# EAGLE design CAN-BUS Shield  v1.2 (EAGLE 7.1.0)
DESCRIPTION: microOBD 200 OBD-II Module; HW_REV: 1.4; PCB_REV: C; PCB_SPEC1: Layer Count: 4; PCB_SPEC2: Size: 1.3" x 0.59"; PCB_SPEC3: Finish Thickness: 0.049" - 0.052"; PCB_SPEC4: Copper Weight: 1oz; TITLE: STM1120

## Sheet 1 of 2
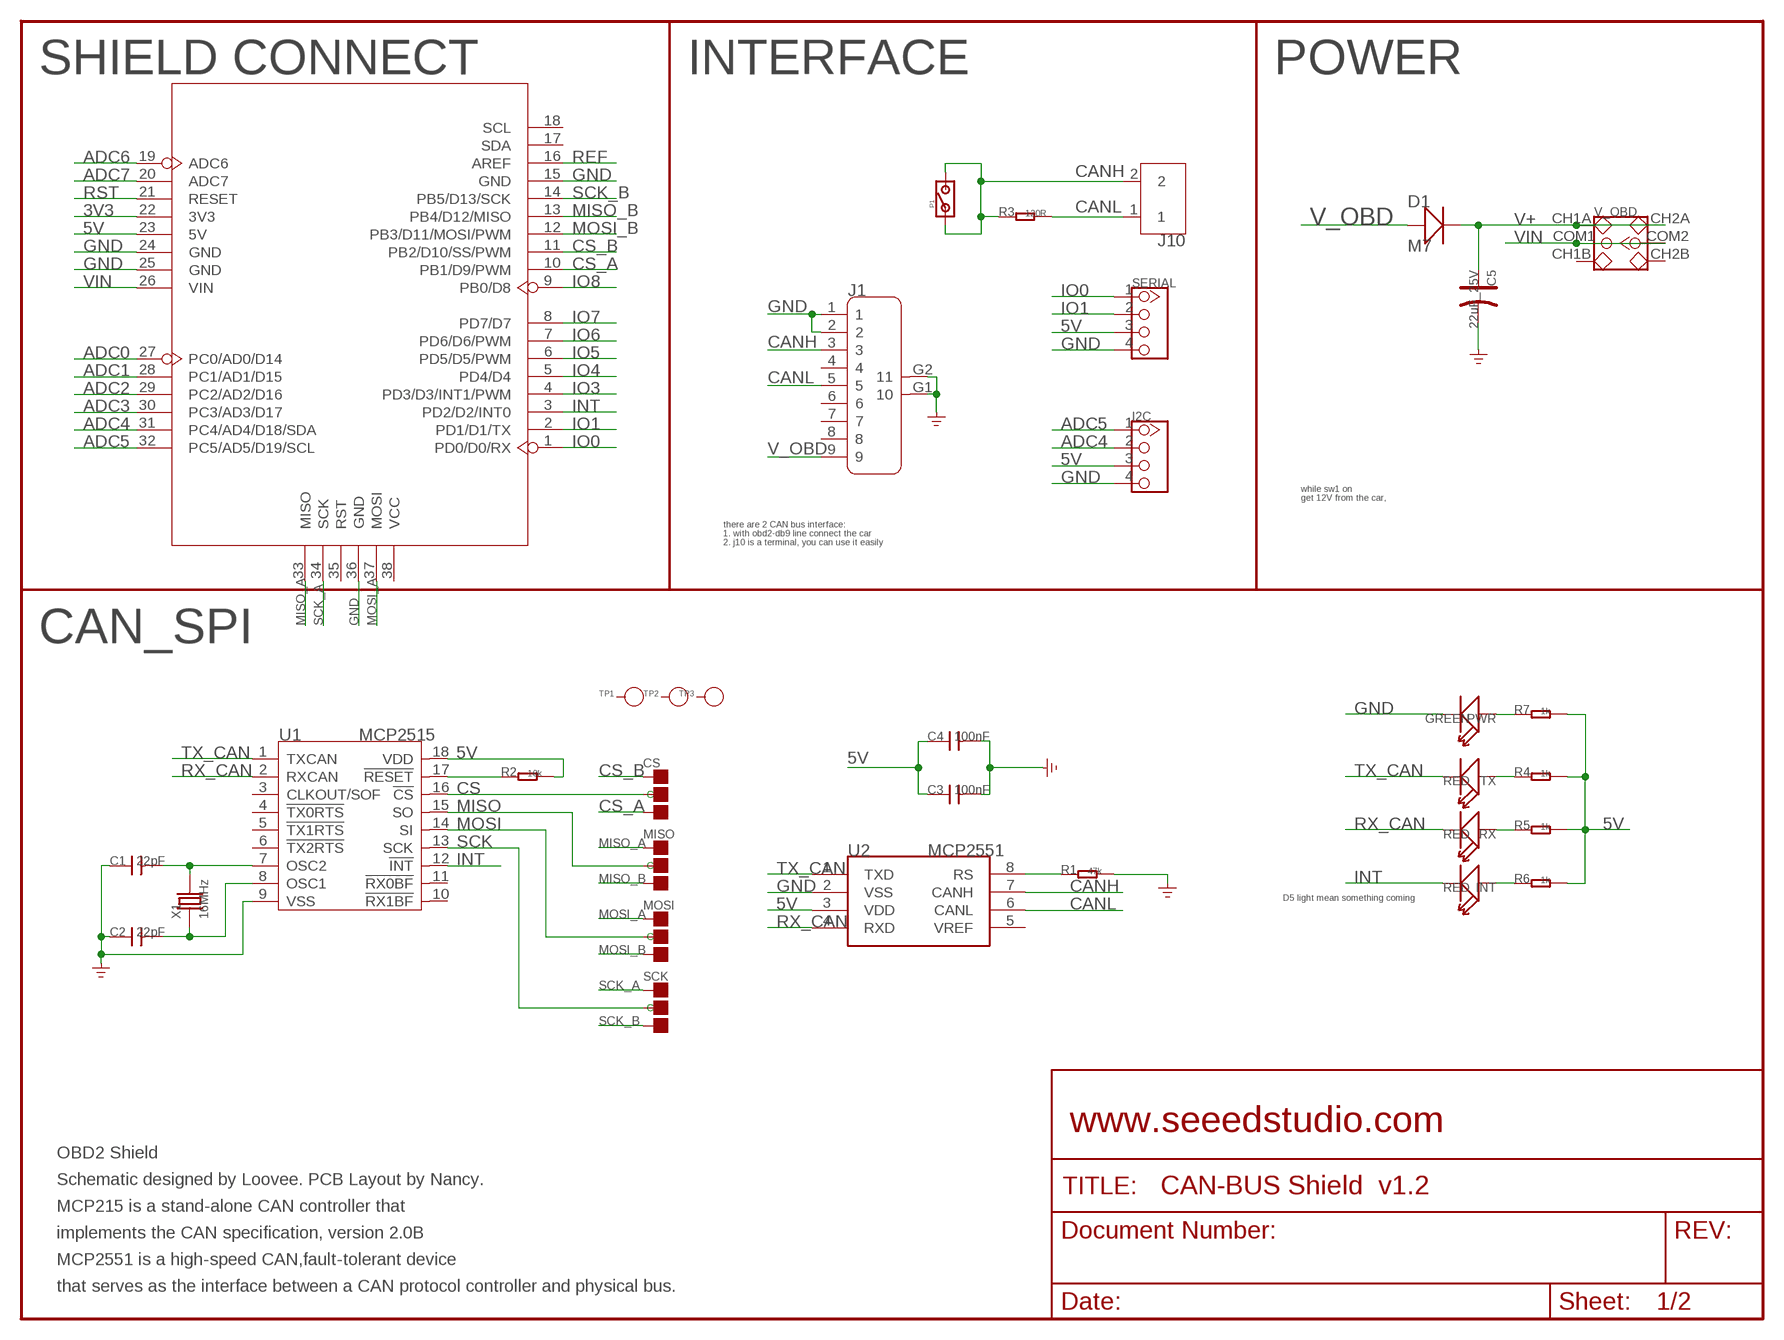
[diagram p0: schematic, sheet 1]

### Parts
C1  22pF  C-0603  [0603]
C2  22pF  C-0603  [0603]
C3  100nF  C-0603  [0603]
C4  100nF  C-0603  [0603]
C5  22uF_25V  CAP-ELECTRO-B  [ELECTRO-SMD-B-4.8MM]
CS  PAD-JUMPER-3P-40*40  [3P-SMD-4.1X1.5]
D1  M7  D-SMA  [D2010]
I2C  TWIG-4P-2.0-2.0  [4P-2.0]
INT  RED  LED'0603'  [LED-0603]
J1  DB9'MEAL'  [DB9-MEAL]
J10  SCREW-TERMINAL-2P5.0  [2P-5.0]
MISO  PAD-JUMPER-3P-40*40  [3P-SMD-4.1X1.5]
MOSI  PAD-JUMPER-3P-40*40  [3P-SMD-4.1X1.5]
P1  PAD-JUMPER-2P  [2P-SMD-1.78X1.27]
PWR  GREEN  LED'0603'  [LED-0603]
R1  47k  R-0603  [0603]
R2  10k  R-0603  [0603]
R3  120R  R-0603  [0603]
R4  1k  R-0603  [0603]
R5  1k  R-0603  [0603]
R6  1k  R-0603  [0603]
R7  1k  R-0603  [0603]
RX  RED  LED'0603'  [LED-0603]
SCK  PAD-JUMPER-3P-40*40  [3P-SMD-4.1X1.5]
SERIAL  TWIG-4P-2.0-2.0  [4P-2.0]
TP1  PAD-TEST-POINT'4545'  [TP_4545]
TP2  PAD-TEST-POINT'4545'  [TP_4545]
TP3  PAD-TEST-POINT'4545'  [TP_4545]
TX  RED  LED'0603'  [LED-0603]
U1  MCP2515  MCP2515-SOIC18  [SOIC18]
U2  MCP2551  MCP2551-SOIC8  [SOIC8-6.0]
U4  ARDUINO-38P'WITH/-SILK'  [ARDUINO-38P-WITH/-SILK-500519002]
V_OBD  SWITCH-2CH-6P  [6P-2CH-2.54-7.6X3.0]
X1  16MHz  CRYSTAL-HC49S  [HC49/S]

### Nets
3V3: U4.22(3V3)
5V: C3.1 C4.1 I2C.3 R2.2 R4.2 R5.2 R6.2 R7.2 SERIAL.3 U1.18(VDD) U2.3(VDD) U4.23(5V)
ADC0: U4.27(PC0/AD0/D14)
ADC1: U4.28(PC1/AD1/D15)
ADC2: U4.29(PC2/AD2/D16)
ADC3: U4.30(PC3/AD3/D17)
ADC4: I2C.2 U4.31(PC4/AD4/D18/SDA)
ADC5: I2C.1 U4.32(PC5/AD5/D19/SCL)
ADC6: U4.19(ADC6)
ADC7: U4.20(ADC7)
CANH: J1.3 J10.2 P1.1 P1.2 R3.1 U2.7(CANH)
CANL: J1.5 J10.1 R3.2 U2.6(CANL)
CS: CS.MM(C) U1.16(!CS)
CS_A: CS.11(R) U4.10(PB1/D9/PWM)
CS_B: CS.00(L) U4.11(PB2/D10/SS/PWM)
GND: C1.1 C2.1 C3.2 C4.2 C5.- I2C.4 J1.1 J1.2 J1.G1 J1.G2 PWR.- R1.2 SERIAL.4 U1.9(VSS) U2.2(VSS) U4.15(GND) U4.24(GND) U4.25(GND) U4.36(GND)
INT: INT.- U1.12(!INT) U4.3(PD2/D2/INT0)
IO0: SERIAL.1 U4.1(PD0/D0/RX)
IO1: SERIAL.2 U4.2(PD1/D1/TX)
IO3: U4.4(PD3/D3/INT1/PWM)
IO4: U4.5(PD4/D4)
IO5: U4.6(PD5/D5/PWM)
IO6: U4.7(PD6/D6/PWM)
IO7: U4.8(PD7/D7)
IO8: U4.9(PB0/D8)
MISO: MISO.MM(C) U1.15(SO)
MISO_A: MISO.00(L) U4.33(MISO)
MISO_B: MISO.11(R) U4.13(PB4/D12/MISO)
MOSI: MOSI.MM(C) U1.14(SI)
MOSI_A: MOSI.00(L) U4.37(MOSI)
MOSI_B: MOSI.11(R) U4.12(PB3/D11/MOSI/PWM)
N$1: PWR.+ R7.1
N$2: R4.1 TX.+
N$15: R5.1 RX.+
N$16: C1.2 U1.7(OSC2) X1.2
N$17: C2.2 U1.8(OSC1) X1.1
N$19: INT.+ R6.1
N$20: R1.1 U2.8(RS)
REF: U4.16(AREF)
RST: U4.21(RESET)
RST_N: R2.1 U1.17(!RESET)
RX_CAN: RX.- U1.2(RXCAN) U2.4(RXD)
SCK: SCK.MM(C) U1.13(SCK)
SCK_A: SCK.00(L) U4.34(SCK)
SCK_B: SCK.11(R) U4.14(PB5/D13/SCK)
TX_CAN: TX.- U1.1(TXCAN) U2.1(TXD)
V+: C5.+ D1.- V_OBD.CH1A V_OBD.CH2A
V_OBD: D1.+ J1.9
VIN: U4.26(VIN) V_OBD.COM1 V_OBD.COM2
Unconnected: J1.4 J1.6 J1.7 J1.8 TP1.T TP2.T TP3.T U1.3(CLKOUT/SOF) U1.4(!TX0RTS) U1.5(!TX1RTS) U1.6(!TX2RTS) U1.10(!RX1BF) U1.11(!RX0BF) U2.5(VREF) U4.17(SDA) U4.18(SCL) U4.35(RST) U4.38(VCC) V_OBD.CH1B V_OBD.CH2B

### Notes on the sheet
- SHIELD CONNECT | INTERFACE | POWER
- while sw1 on
- get 12V from the car,
- there are 2 CAN bus interface:
- 1. with obd2-db9 line connect the car
- 2. j10 is a terminal, you can use it easily
- CAN_SPI
- D5 light mean something coming
- www.seeedstudio.com
- OBD2 Shield
- Schematic designed by Loovee. PCB Layout by Nancy.
- MCP215 is a stand-alone CAN controller that
- implements the CAN specification, version 2.0B
- MCP2551 is a high-speed CAN,fault-tolerant device
- that serves as the interface between a CAN protocol controller and physical bus.

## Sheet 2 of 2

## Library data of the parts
C1-C4 = Discrete:C*: Ceramic Capacitors
C5 = Discrete:CAP*: Electrolytic Capacitors,Tantalum Capacitors and Super Capacitors
CS MISO MOSI SCK = Discrete:PAD-JUMPER-3P
D1 = Discrete:D*
I2C SERIAL = Connector:TWIG-4P-2.0
INT PWR RX TX = Discrete:LED*
J1 = Connector:DB9
J10 = Connector:SCREW-TERMINAL-2P
P1 = Discrete:PAD-JUMPER-2P
R1-R7 = Discrete:R*
TP1-TP3 = Discrete:PAD-TEST-POINT; PARTNO: DNP
U1 = IC:MCP2515: Stand-Alone CAN Controller With SPI Interface
U2 = IC:MCP2551: High-Speed CAN Transceiver http://ww1.microchip.com/downloads/en/devicedoc/21667f.pdf
U4 = moudle:ARDUINO-38P
V_OBD = Discrete:SWITCH-2CH-6P
X1 = Discrete:CRYSTAL*: CRYSTAL

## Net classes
0 default: width 0.152 mm, drill 0.305 mm, clearance 0.152 mm

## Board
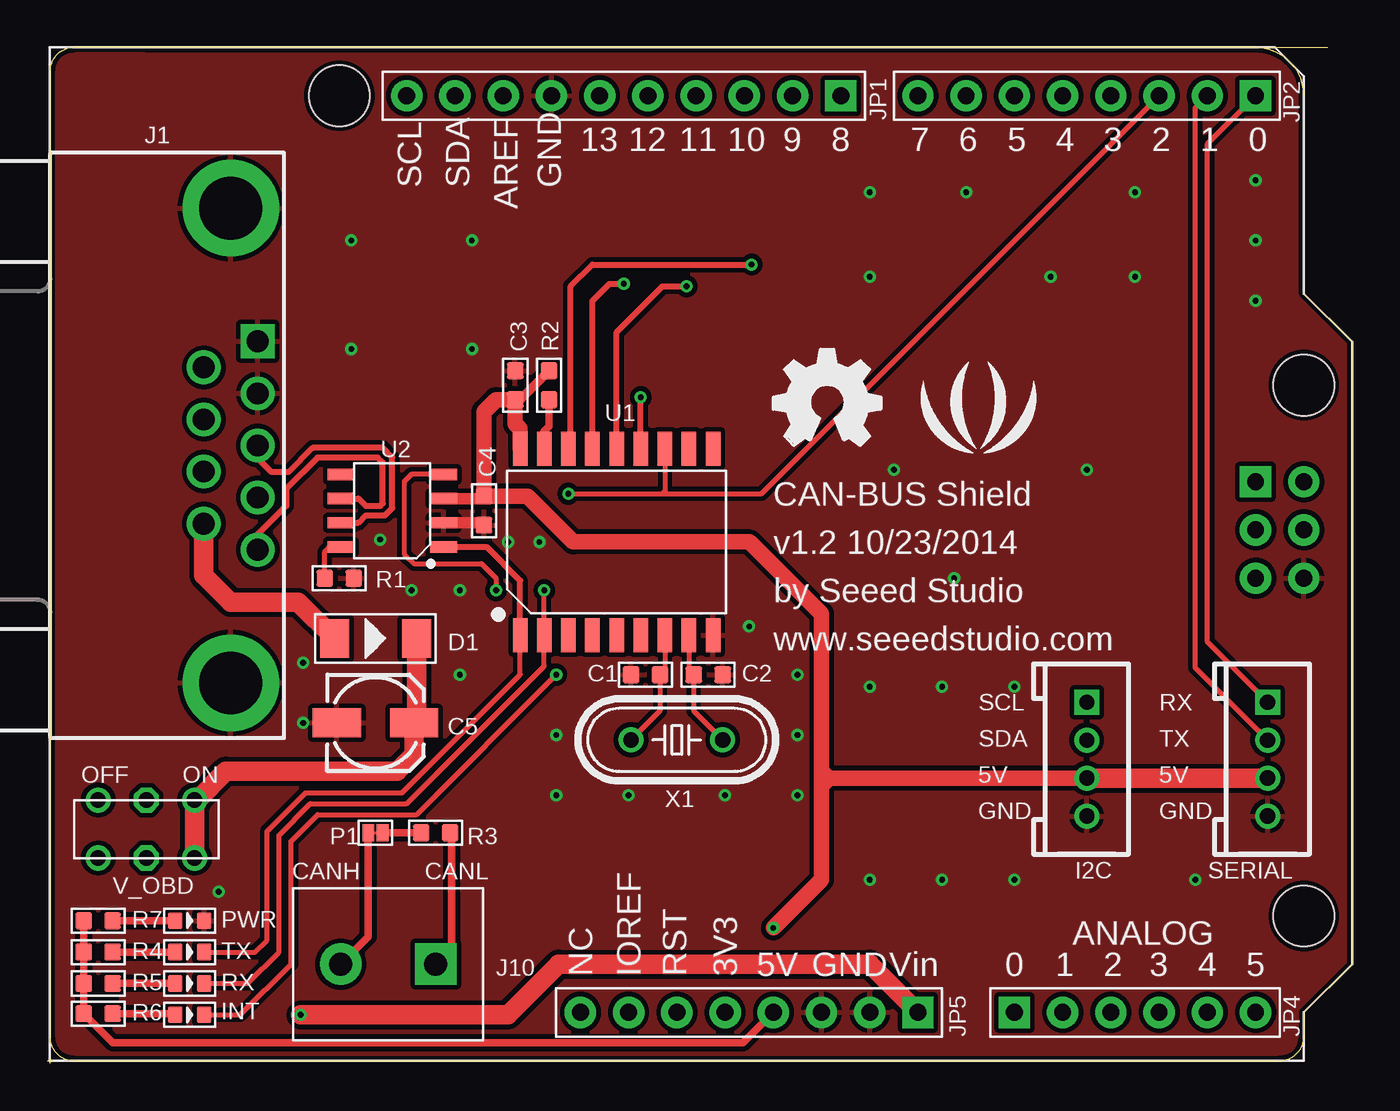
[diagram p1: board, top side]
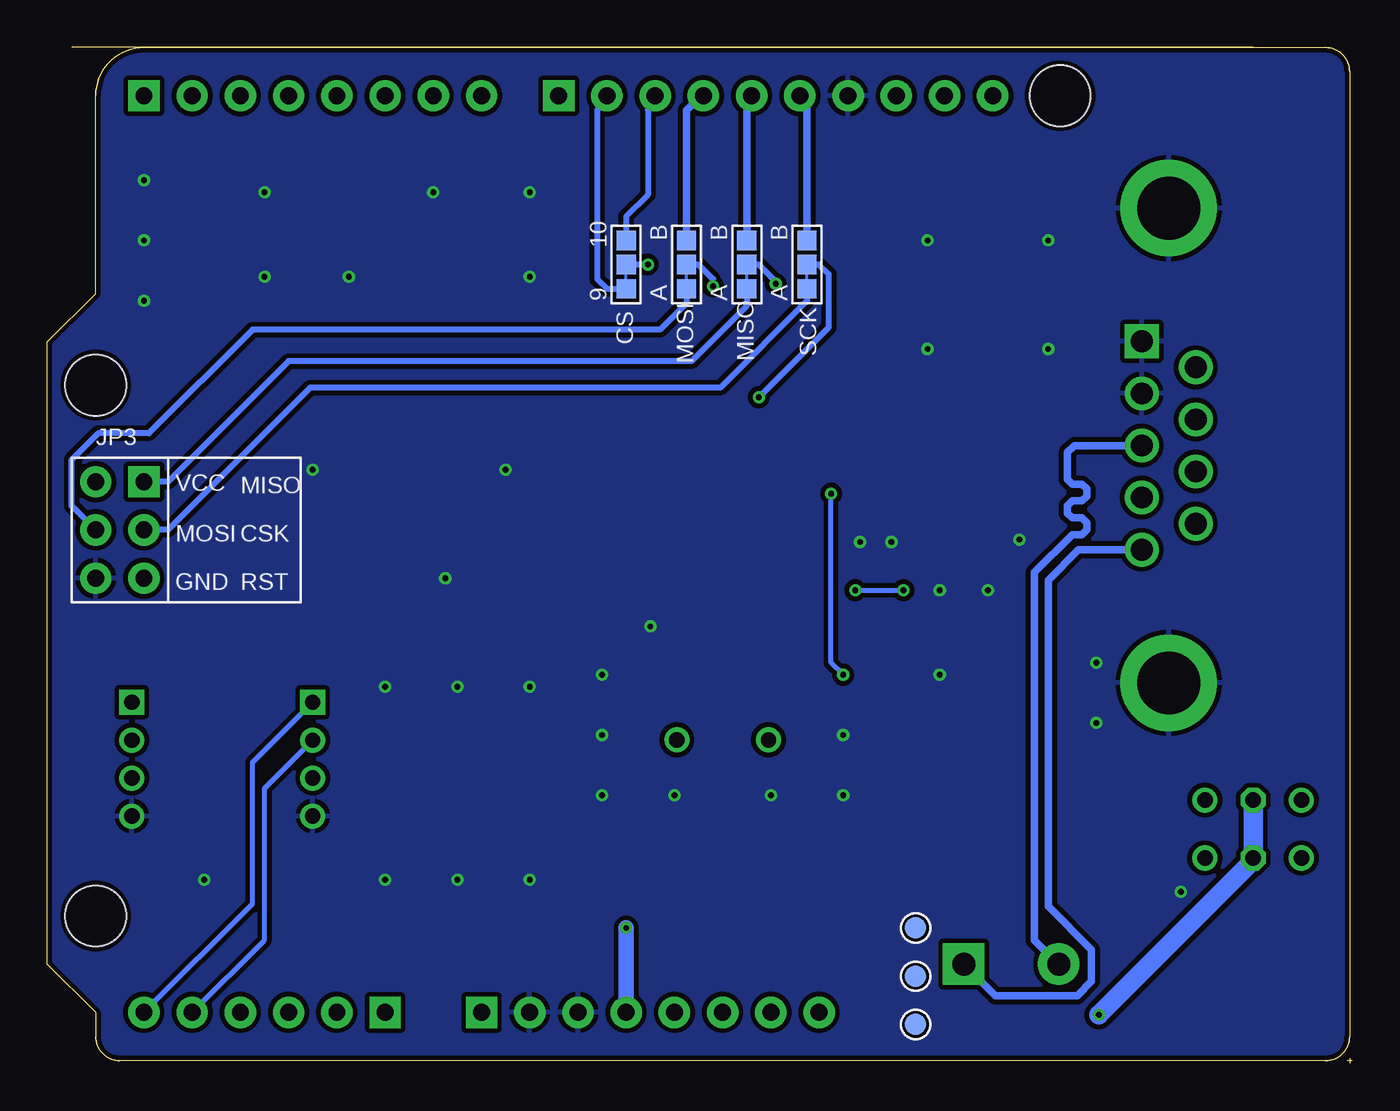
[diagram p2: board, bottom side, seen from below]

Size 68.71 x 53.47 mm. Coordinates in mm from the lower left corner, seen from the top.
Outline: 66.17,1.4 arc-90 64.9,0.13
Outline: 1.4,0.13 arc-90 0.13,1.4
Outline: 0.13,52.2 arc-90 1.4,53.47
Outline: 63.63,53.47 arc-90 66.17,50.93
Outline: 5.21,53.47 67.44,53.47
Outline: 0.13,1.4 arc90 1.4,0.13
Outline: 64.9,0.13 arc90 66.17,1.4
Outline: 1.4,53.47 arc90 0.13,52.2
Outline: 0.13,1.4 arc90 1.4,0.13
Outline: 64.9,0.13 arc90 66.17,1.4
Outline: 66.17,50.93 arc90 63.63,53.47
Outline: 66.17,1.4 66.17,2.67 68.71,5.21 68.71,37.97 66.17,40.51 66.17,50.93
Outline: 66.17,1.4 arc-90 64.9,0.13
Outline: 63.63,53.47 1.4,53.47
Outline: 1.4,53.47 arc90 0.13,52.2
Outline: 0.13,52.2 0.13,1.4
Outline: 0.13,1.4 arc90 1.4,0.13
Outline: 66.17,50.93 arc90 63.63,53.47
Outline: 1.4,0.13 64.9,0.13
Outline: 0,0.13 0.25,0.13
Outline: 0.13,0.25 0.13,0
Copper layers (1*16): Top 0.035mm / dielectric 1.5mm / Bottom 0.035mm
Design rules "SeeedStudio_2layer_DRU_no_angle_20140221 *": minimum track width 6mil, minimum drill 12mil, track to track 6mil, track to pad 6mil, pad to pad 6mil, via to via 6mil, smd to smd 0mil, copper to edge 10mil, drill to drill 10mil, minimum pad ring 10mil, minimum via ring 6mil, stop-mask expansion 2mil, vias tented up to drill 100mil, thermal gap 10mil

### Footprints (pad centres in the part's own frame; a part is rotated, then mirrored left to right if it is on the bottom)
0603 = smd 0.889 x 0.889: 1 -0.762,0; 2 0.762,0
ELECTRO-SMD-B-4.8MM = smd 2.54 x 1.524: + 2.032,0; - -2.032,0
3P-SMD-4.1X1.5 = smd 1.016 x 1.016: 00 -1.27,0; 11 1.27,0; MM 0,0
D2010 = smd 1.524 x 2.032: + -2.159,0; - 2.159,0
4P-2.0 = drill 0.8 pad 1.27 square: 1 -3,0 | drill 0.8 pad 1.27: 2 -1,0; 3 1,0; 4 3,0
LED-0603 = smd 0.762 x 0.889: + -0.762,0; - 0.762,0
DB9-MEAL = drill 1.143 pad 1.778 square: 1 -5.486,1.422 | drill 1.143 pad 1.778: 2 -2.743,1.422; 3 0,1.422; 4 2.743,1.422; 5 5.486,1.422; 6 -4.115,-1.422; 7 -1.372,-1.422; 8 1.372,-1.422; 9 4.115,-1.422 | drill 3.302 pad 5.08: G1 12.497,0; G2 -12.497,0
2P-5.0 = drill 1.2 pad 2.184 square: 1 0,0 | drill 1.2 pad 2.184: 2 5,0
2P-SMD-1.78X1.27 = smd 0.889 x 0.61: 1 0,0.381; 2 0,-0.381
TP_4545 = smd 1.143 x 1.143: T 0,0
SOIC18 = smd 0.762 x 1.778: 1 -5.08,-4.915; 2 -3.81,-4.915; 3 -2.54,-4.915; 4 -1.27,-4.915; 5 0,-4.915; 6 1.27,-4.915; 7 2.54,-4.915; 8 3.81,-4.915; 9 5.08,-4.915; 10 5.08,4.915; 11 3.81,4.915; 12 2.54,4.915; 13 1.27,4.915; 14 0,4.915; 15 -1.27,4.915; 16 -2.54,4.915; 17 -3.81,4.915; 18 -5.08,4.915
SOIC8-6.0 = smd 0.6 x 1.4: 1 -1.905,-2.7; 2 -0.635,-2.7; 3 0.635,-2.7; 4 1.905,-2.7; 5 1.905,2.7; 6 0.635,2.7; 7 -0.635,2.7; 8 -1.905,2.7
ARDUINO-38P-WITH/-SILK-500519002 = drill 0.889 pad 1.651 square: 1 63.5,50.8; 9 41.656,50.8; 26 45.72,2.54; 27 50.8,2.54; 33 63.5,30.48 | drill 0.889 pad 1.651: 2 60.96,50.8; 3 58.42,50.8; 4 55.88,50.8; 5 53.34,50.8; 6 50.8,50.8; 7 48.26,50.8; 8 45.72,50.8; 10 39.116,50.8; 11 36.576,50.8; 12 34.036,50.8; 13 31.496,50.8; 14 28.956,50.8; 15 26.416,50.8; 16 23.876,50.8; 17 21.336,50.8; 18 18.796,50.8; 19 27.94,2.54; 20 30.48,2.54; 21 33.02,2.54; 22 35.56,2.54; 23 38.1,2.54; 24 40.64,2.54; 25 43.18,2.54; 28 53.34,2.54; 29 55.88,2.54; 30 58.42,2.54; 31 60.96,2.54; 32 63.5,2.54; 34 63.5,27.94; 35 63.5,25.4; 36 66.04,25.4; 37 66.04,27.94; 38 66.04,30.48 | hole 3.2: 15.24,50.8; 66.04,35.56; 66.04,7.62
6P-2CH-2.54-7.6X3.0 = drill 0.813 pad 1.27: CH1A -1.524,2.54; CH1B -1.524,-2.54; CH2A 1.524,2.54; CH2B 1.524,-2.54 | drill 0.813 pad 1.27 octagon: COM1 -1.524,0; COM2 1.524,0
HC49/S = drill 0.813: 1 -2.413,0; 2 2.413,0

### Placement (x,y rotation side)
C1  31.5,20.45 0 top
C2  34.8,20.45 180 top
C3  24.64,35.69 90 top
C4  22.99,29.08 270 top
C5  17.27,17.91 0 top
CS  38.23,42.04 270 bottom
D1  17.27,22.35 0 top
I2C  54.74,16 270 top
INT  7.49,2.54 0 top
J1  9.65,32.51 270 top
J10  20.45,5.21 180 top
MISO  31.88,42.04 90 bottom
MOSI  35.05,42.04 90 bottom
P1  17.27,12.13 90 top
PWR  7.49,7.49 0 top
R1  15.37,25.53 0 top
R2  26.42,35.69 90 top
R3  20.45,12.13 0 top
R4  2.67,5.84 180 top
R5  2.67,4.19 180 top
R6  2.67,2.6 180 top
R7  2.67,7.49 180 top
RX  7.49,4.19 0 top
SCK  28.7,42.04 90 bottom
SERIAL  64.26,16 270 top
TP1  22.99,7.11 0 bottom
TP2  22.99,4.57 0 bottom
TP3  22.99,2.03 0 bottom
TX  7.49,5.84 0 top
U1  29.97,27.43 0 top
U2  18.16,29.08 90 top
U4  0.13,0.13 0 top
U$1  [LOGO_SILK]  49.02,33.78 0 top
U$2  [OSHW_FILLX200_NOTEXT]  38.23,32.51 0 top
V_OBD  5.21,12.32 270 top
X1  33.15,17.02 180 top

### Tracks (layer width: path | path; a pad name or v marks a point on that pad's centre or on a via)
5V  (via drill 0.3 pad 0.64)
  Top 0.254: R4.2 1.91,5.71
  Top 0.406: 1.91,5.71 R5.2 R6.2 3.43,1.08 36.64,1.08 U4.23 | R4.2 R7.2
  Top 0.508: C3.1 24.89,34.93 R2.2
  Top 0.61: U2.3 23.11,29.72 C4.1
  Top 0.813: 40.77,15.37 40.77,23.64 36.98,27.43 27.69,27.43 25.27,29.84 C4.1 22.99,34.29 23.62,34.93 C3.1 24.64,33.66 24.89,33.4 U1.18 | 40.77,15.37 40.77,15.11 | 40.77,15.11 40.77,14.61 | I2C.3 41.16,15 | 41.13,15 40.88,15 40.77,15.11 | 41.16,15 41.13,15 | 41.13,15 40.77,15.37 | 41.16,15 40.77,14.61 | 40.77,14.61 40.77,9.65 v38.23,7.11
  Top 1.016: I2C.3 SERIAL.3
  Bottom 0.813: v38.23,7.11 U4.23
ADC4
  Bottom 0.254: U4.31 57.28,6.48 57.28,14.46 I2C.2
ADC5
  Bottom 0.254: U4.32 57.91,8.38 57.91,15.83 I2C.1
CANH
  Top 0.152: P1.1 P1.2
  Top 0.305: U2.7 16.38,28.45 16.76,28.83 17.78,28.83 18.16,29.21 18.16,31.88 17.65,32.39 13.97,32.39 12.7,31.11 11.81,31.11 11.07,31.85 J1.3
  Top 0.406: P1.1 16.89,6.65 J10.2 | R3.1 P1.2
  Bottom 0.406: 11.05,32.51 J1.3 14.63,32.51 14.99,32.15 14.99,30.73 14.73,30.48 14.22,30.48 13.97,30.23 13.97,29.84 14.22,29.59 14.73,29.59 14.99,29.34 14.99,28.96 14.73,28.7 14.22,28.7 13.97,28.45 13.97,28.07 14.22,27.81 14.73,27.81 16.72,25.83 16.72,6.48 J10.2
CANL
  Top 0.305: U2.6 16.38,29.72 16.76,29.34 17.53,29.34 17.65,29.46 17.65,31.62 17.4,31.88 14.22,31.88 12.57,30.23 12.57,29.34 11.07,27.84 J1.5
  Top 0.406: R3.2 21.27,12.13 21.27,6.03 J10.1
  Bottom 0.406: J1.5 14.4,27.03 16,25.43 16,8.26 13.72,5.97 13.72,4.32 14.48,3.56 18.8,3.56 J10.1
CS  (via drill 0.3 pad 0.64)
  Top 0.305: U1.16 27.43,33.02 27.56,33.15 27.56,40.89 28.7,42.04 v37.08,42.04
  Bottom 0.305: v37.08,42.04 CS.MM
CS_A
  Bottom 0.152: CS.11 38.23,42.04
  Bottom 0.305: U4.10 39.24,50.67 39.75,50.16 39.75,41.28 39.24,40.77 CS.11
CS_B
  Bottom 0.305: U4.11 36.7,50.55 37.08,50.16 37.08,45.72 38.23,44.58 CS.00
GND  (via drill 0.3 pad 0.64)
  Top 0.61: U2.2 22.86,28.45 C4.2
  other vias: 24.26,27.43 17.53,27.56 25.91,27.43 13.46,17.91 21.72,24.89 19.18,24.89 9.02,9.02 26.8,17.27 26.8,14.1 30.61,14.1 39.5,17.27 39.5,20.45 36.96,22.99 35.69,14.1 39.5,14.1 16,43.31 22.35,43.31 16,37.59 22.35,37.59 43.31,41.4 57.28,45.85 57.28,41.4 63.63,46.48 63.63,40.13 43.31,45.85 43.31,9.65 47.12,9.65 50.93,9.65 43.31,19.81 47.12,19.81 50.93,19.81 54.74,31.24 44.58,31.24 47.75,25.53 48.39,45.85 60.45,9.65 52.83,41.4 63.63,43.31 13.46,21.08 21.72,20.45
  pour Top (isolate 0.254): 0.13,53.47 68.71,53.47 68.71,0.13 0.13,0.13
  pour Bottom (isolate 0.254): 0.13,53.47 68.71,53.47 68.71,0.13 0.13,0.13
INT  (via drill 0.3 pad 0.64)
  Top 0.254: INT.- 10.16,2.54 12.83,5.21 12.83,11.68 14.22,13.08 19.43,13.08 v26.8,20.45 | U1.12 32.51,29.97 | 32.64,29.97 37.59,29.97 U4.3 | v27.43,29.97 32.39,29.97 | 32.39,29.97 32.51,29.97 | 32.51,29.97 32.64,29.97 | 32.39,29.97 32.51,30.1 32.64,29.97
  Bottom 0.254: v26.8,20.45 27.43,21.08 v27.43,29.97
IO0
  Top 0.254: SERIAL.1 61.09,22.18 61.09,48.39 U4.1
IO1
  Top 0.254: SERIAL.2 60.45,20.81 60.45,50.29 U4.2
MISO  (via drill 0.3 pad 0.64)
  Top 0.305: U1.15 28.7,40.13 29.59,41.02 v30.35,41.02
  Bottom 0.305: v30.35,41.02 30.35,41.15 31.24,42.04 MISO.MM 31.75,41.91
MISO_A
  Bottom 0.152: MISO.00 31.88,42.04
  Bottom 0.305: MISO.00 31.88,39.88 34.8,36.96 56.01,36.96 62.36,30.61 U4.33
MISO_B
  Bottom 0.406: U4.13 31.62,50.8 31.88,50.55 MISO.11
MOSI  (via drill 0.3 pad 0.64)
  Top 0.305: U1.14 29.97,38.48 32.39,40.89 v33.66,40.89
  Bottom 0.305: v33.66,40.89 33.66,41.28 34.42,42.04 MOSI.MM
MOSI_A
  Bottom 0.152: MOSI.00 35.05,42.04
  Bottom 0.305: MOSI.00 35.05,40.01 36.45,38.61 57.91,38.61 63.37,33.15 66.04,33.15 67.44,31.75 67.44,29.34 U4.37
MOSI_B
  Bottom 0.406: U4.12 34.29,50.93 35.05,50.16 MOSI.11
N$1
  Top 0.406: R7.1 PWR.+
N$2
  Top 0.406: R4.1 TX.+
N$15
  Top 0.406: R5.1 RX.+
N$16
  Top 0.254: U1.7 32.51,20.7 C1.2 32.26,18.54 X1.2
N$17
  Top 0.254: U1.8 33.78,20.7 C2.2 34.04,18.54 X1.1
N$19
  Top 0.406: R6.1 6.67,2.6 INT.+
N$20
  Top 0.254: R1.1 14.61,26.92 14.86,27.18 U2.8 15.56,27.18
RST_N
  Top 0.406: R2.1 26.42,33.53 26.16,33.27 U1.17
RX_CAN  (via drill 0.3 pad 0.64)
  Top 0.254: RX.- 10.54,4.19 12.19,5.84 12.19,12 13.84,13.65 18.92,13.65 26.16,20.89 U1.2 v26.16,24.89 | U2.4 19.18,30.99 18.8,30.61 18.8,26.8 19.3,26.29 22.86,26.29 23.62,25.53 v23.62,24.89
  Bottom 0.254: v26.16,24.89 v23.62,24.89
SCK  (via drill 0.3 pad 0.64)
  Top 0.305: U1.13 v31.24,35.05
  Bottom 0.305: v31.24,35.05 31.24,35.18 31.11,35.18 27.56,38.73 27.56,41.53 28.07,42.04 SCK.MM
SCK_A
  Bottom 0.152: SCK.00 28.7,42.04
  Bottom 0.305: SCK.00 28.7,40.13 33.27,35.56 54.86,35.56 62.36,28.07 U4.34
SCK_B
  Bottom 0.406: U4.14 28.7,50.55 SCK.11
TX_CAN
  Top 0.254: TX.- 10.92,5.84 11.56,6.48 11.56,12.19 13.59,14.22 18.67,14.22 24.89,20.45 U1.1
  Top 0.305: U2.1 23.11,27.18 24.89,25.4 U1.1
V+
  Top 1.016: V_OBD.CH2A V_OBD.CH1A 7.87,13.84 9.4,15.37 18.41,15.37 19.3,16.26 19.3,17.65 | C5.+ 19.3,17.65 | D1.- 19.43,17.78 19.3,17.65
V_OBD
  Top 1.016: J1.9 8.23,25.68 9.65,24.26 13.21,24.26 D1.+
VIN  (via drill 0.3 pad 0.64)
  Top 1.016: v13.34,2.54 24.26,2.54 26.92,5.21 43.31,5.21 U4.26
  Bottom 1.016: V_OBD.COM1 V_OBD.COM2 5.21,10.67 v13.34,2.54

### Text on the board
tPlace: CAN-BUS Shield | v1.2 10/23/2014 | by Seeed Studio | www.seeedstudio.com | SCL | RX | SDA | TX | OFF | ON | 5V | 5V | GND | GND | CANH | CANL
bPlace: B | B | B | 10 | A | A | A | 9 | MISO | VCC | CSK | MOSI | RST | GND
